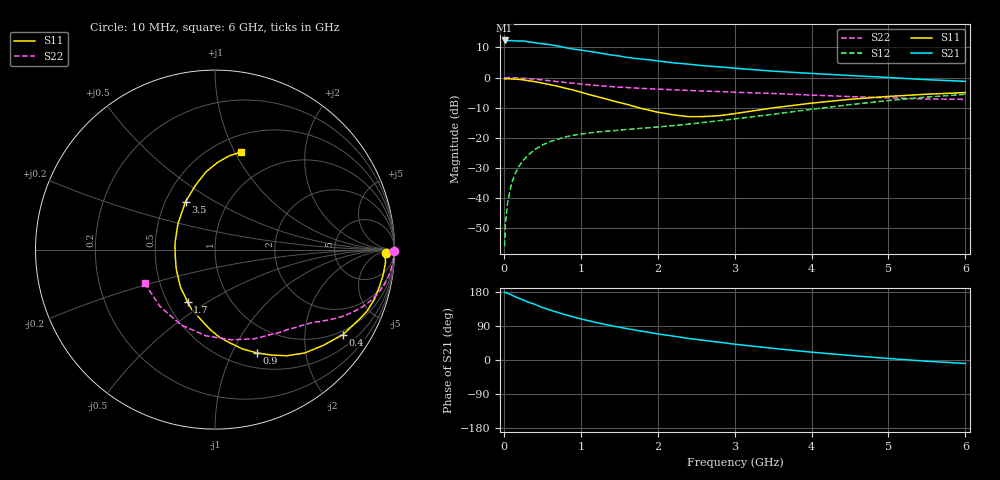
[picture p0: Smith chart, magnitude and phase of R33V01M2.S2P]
! SIEMENS Small Signal Semiconductors
! BFR181
! Si NPN RF Bipolar Junction Transistor in SOT23
! VCE = 3 V  IC = 1.2 mA
! Common Emitter S-Parameters:  May  1996
# GHz  S  MA  R  50
!  f  S11  S21  S12  S22
! GHz  MAG  ANG  MAG  ANG  MAG  ANG  MAG  ANG
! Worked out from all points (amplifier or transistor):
!   36 points, 10 MHz to 6 GHz, reference 50 ohm
!   highest |S21| = 12.3 dB at 10 MHz (marker M1)
!   |S21| within 3 dB of that: start of sweep to 944.6 MHz
!   unconditionally stable (mu >= 1): 1.923 GHz to 3.613 GHz
!   at 250 MHz: K = 0.18, MSG = 19.8 dB, |S12| = -27.5 dB
!   at 1.4 GHz: K = 0.82, MSG = 12.6 dB, |S12| = -17.7 dB
!   at 6 GHz: K = 0.87, MSG = 2.2 dB, |S12| = -5.6 dB
!   S11 on the Smith chart (normalised r, x): 10 MHz: 36, -13; 400 MHz: 0.87, -3.09; 900 MHz: 0.67, -1.25; 1.7 GHz: 0.63, -0.41; 3.5 GHz: 0.63, +0.38; 6 GHz: 0.67, +1.06
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0.01  0.952 -1.0  4.114 179.4  0.0016 96.0  0.9988 -0.4
0.02  0.9468 -2.0  4.058 178.1  0.0036 94.4  0.9886 -0.8
0.05  0.953 -4.1  4.059 175.8  0.0086 87.1  0.9976 -2.0
0.1  0.9476 -8.6  4.106 171.8  0.0175 84.7  0.9953 -4.0
0.15  0.9381 -13.0  4.037 166.6  0.0259 81.3  0.9872 -6.2
0.25  0.9149 -21.8  4.042 158.3  0.042 75.5  0.9726 -10.0
0.3  0.8932 -25.7  3.946 154.1  0.0495 74.0  0.9621 -11.9
0.4  0.8559 -33.6  3.768 147.1  0.0636 69.1  0.9391 -15.2
0.5  0.8048 -41.6  3.63 138.6  0.0759 64.9  0.9118 -18.3
0.6  0.7627 -49.0  3.499 131.8  0.0864 61.1  0.8814 -21.2
0.7  0.7151 -55.8  3.322 125.6  0.0951 57.8  0.8532 -23.5
0.9  0.6207 -68.0  2.963 113.7  0.1104 52.7  0.8053 -27.4
1.1  0.525 -81.1  2.726 103.6  0.1201 49.4  0.7606 -30.6
1.4  0.416 -98.2  2.36 90.4  0.1306 46.8  0.7071 -34.6
1.7  0.3302 -117.6  2.081 79.3  0.1408 46.5  0.6695 -37.7
2  0.2663 -138.9  1.883 68.9  0.1515 47.4  0.6423 -41.1
2.2  0.2407 -153.9  1.751 63.1  0.1593 48.3  0.6265 -43.7
2.8  0.2331 157.2  1.502 46.9  0.1921 51.4  0.5853 -52.1
3.5  0.3138 121.5  1.275 30.7  0.2461 52.2  0.5436 -66.0
4.5  0.4354 96.7  1.079 11.9  0.3549 46.5  0.4831 -95.9
5.5  0.5289 81.3  0.92 -3.2  0.4737 34.0  0.4408 -134.2
6  0.5628 75.0  0.864 -9.2  0.5264 26.3  0.4347 -154.6
